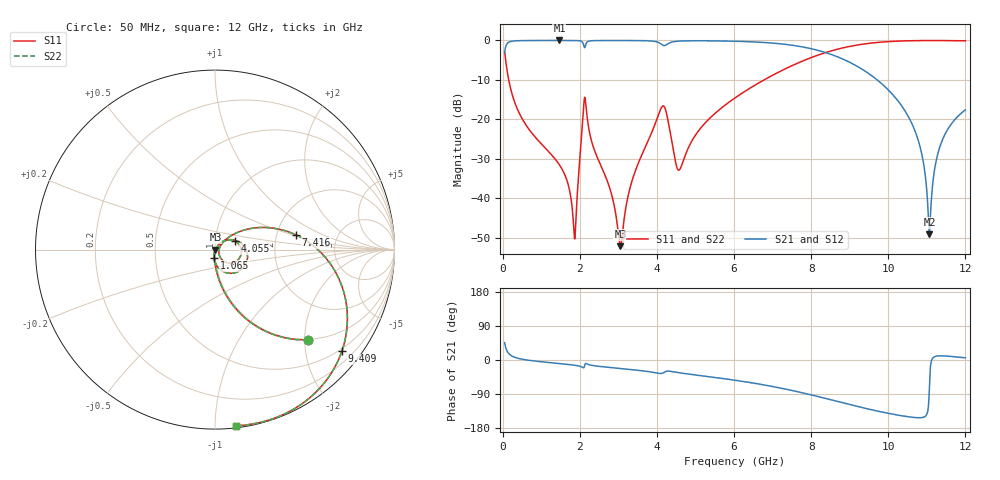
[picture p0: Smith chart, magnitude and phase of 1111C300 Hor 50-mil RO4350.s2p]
# GHz S MA R 50
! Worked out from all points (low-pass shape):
!   11951 points, 50 MHz to 12 GHz, reference 50 ohm
!   highest |S21| = -0.01 dB at 1.473 GHz (marker M1); lowest = -49.1 dB at 11.07 GHz (marker M2)
!   |S21| within 3 dB of the highest: 52.09 MHz to 8.35 GHz (8.298 GHz wide, 198 % of centre)
!   lowest |S11| = -52.1 dB at 3.053 GHz (marker M3), VSWR 1.00, Z = 50.2 - j0.1 ohm
!   |S11| at or under -10 dB: 156.2 MHz to 6.78 GHz (6.624 GHz wide, 191 % of centre)
!   |S22| runs from -52.1 to 0.0 dB; largest |S21 - S12| = 0
!   S11 on the Smith chart (normalised r, x): 50 MHz: 0.99, -2.07; 1.065 GHz: 0.99, -0.09; 4.055 GHz: 1.24, +0.12; 7.416 GHz: 2.55, +0.53; 9.409 GHz: 0.44, -2.78; 12 GHz: 0.01, -1.13
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0.05  0.7214 -44.2  0.6923 45.8  0.6923 45.8  0.7214 -44.2
0.239  0.2126 -79.4  0.9767 10.5  0.9767 10.5  0.2126 -79.4
1.065  0.04534 -94.4  0.9982 -5.3  0.9982 -5.3  0.04534 -94.4
1.473  0.02644 -97.3  0.9986 -9.4  0.9986 -9.4  0.02644 -97.3
1.862  0.003115 -34.7  0.997 -13.7  0.997 -13.7  0.003115 -34.7
2.042  0.05577 46.8  0.9748 -18.0  0.9748 -18.0  0.05577 46.8
2.151  0.1637 -53.7  0.8762 -9.3  0.8762 -9.3  0.1637 -53.7
3.053  0.002471 -23.8  0.9973 -22.4  0.9973 -22.4  0.002471 -23.8
3.358  0.01683 53.2  0.9964 -25.5  0.9964 -25.5  0.01683 53.2
4.034  0.112 28.0  0.944 -35.1  0.944 -35.1  0.112 28.0
4.055  0.1195 24.1  0.9337 -35.4  0.9337 -35.4  0.1195 24.1
4.219  0.1343 -29.3  0.8655 -30.8  0.8655 -30.8  0.1343 -29.3
4.574  0.02268 -5.3  0.9797 -33.7  0.9797 -33.7  0.02268 -5.3
6.025  0.1868 34.7  0.9758 -53.4  0.9758 -53.4  0.1868 34.7
7.416  0.4572 10.4  0.8804 -78.5  0.8804 -78.5  0.4572 10.4
8.017  0.6098 -3.4  0.7817 -92.4  0.7817 -92.4  0.6098 -3.4
9.409  0.906 -38.7  0.4052 -127.6  0.4052 -127.6  0.906 -38.7
10.009  0.966 -52.3  0.2336 -140.9  0.2336 -140.9  0.966 -52.3
10.752  0.9937 -66.2  0.05926 -152.3  0.05926 -152.3  0.9937 -66.2
11.066  0.996 -71.2  0.003502 -70.8  0.003502 -70.8  0.996 -71.2
11.354  0.9954 -75.3  0.0473 11.0  0.0473 11.0  0.9954 -75.3
12  0.9886 -83.2  0.1319 5.8  0.1319 5.8  0.9886 -83.2
